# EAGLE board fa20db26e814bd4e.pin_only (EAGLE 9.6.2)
REV: C

Size 25.4 x 17.78 mm. Coordinates in mm from the lower left corner, seen from the top.
Outline: 0,15.24 0,2.54 arc90 2.54,0 22.86,0 arc90 25.4,2.54 25.4,15.24 arc90 22.86,17.78 2.54,17.78 arc90 0,15.24
Copper layers (1*16): Top 0.035mm / dielectric 1.5mm / Bottom 0.035mm
Design rules "adafruit *": minimum track width 7mil, minimum drill 15.5mil, track to track 7mil, track to pad 7mil, pad to pad 7mil, via to via 7mil, smd to smd 7mil, copper to edge 10mil, drill to drill 8mil, minimum pad ring 10mil, minimum via ring 8mil, stop-mask expansion 2mil, vias tented up to drill 20mil, thermal gap 10mil
Net classes: 1 highpower: width 0.406 mm, drill 0.483 mm; 2 lowpower: width 0.305 mm, drill 0.483 mm
tRestrict: area 11.6,7.9 to 13.5,9.9
bRestrict: area 11.1,7.4 to 14,10.4

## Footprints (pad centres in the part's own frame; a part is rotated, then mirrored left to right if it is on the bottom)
0603-NO = smd 1.075 x 1: 1 -0.85,0; 2 0.85,0
0805-NO = smd 1.24 x 1.5: 1 -0.95,0; 2 0.95,0
JST_SH4 = smd 0.6 x 1.55: 1 -1.5,2.514; 2 -0.5,2.514; 3 0.5,2.514; 4 1.5,2.514 | smd 1.2 x 1.8: MT1 -2.8,-1.386; MT2 2.8,-1.386
CHIPLED_0603_NOOUTLINE = smd 0.8 x 0.8: A 0,-0.75; C 0,0.75
SOD-323_MINI = smd 0.9 x 0.8: A 1.07,0; C -1.07,0
FIDUCIAL_1MM = smd 1 x 1: 1 0,0
1X06_ROUND_70 = drill 1 pad 1.778: 1 -6.35,0; 2 -3.81,0; 3 -1.27,0; 4 1.27,0; 5 3.81,0; 6 6.35,0
SOT363 = smd 0.5 x 0.5: 1 -0.75,-0.9; 3 0.75,-0.9; 4 0.75,0.9; 6 -0.75,0.9 | smd 0.4 x 0.5: 2 0,-0.9; 5 0,0.9
RESPACK_4X0603 = smd 0.45 x 0.9: 1 -1.3,-0.85; 2 -0.4,-0.85; 3 0.4,-0.85; 4 1.3,-0.85; 5 1.3,0.85; 6 0.4,0.85; 7 -0.4,0.85; 8 -1.3,0.85
SOLDERJUMPER_ARROW_NOPASTE = smd 0.762 x 1.524: 1 -1.016,0; 2 1.016,0
SOT23-5 = smd 0.55 x 1.2: 1 -0.95,-1.3; 2 0,-1.3; 3 0.95,-1.3; 4 0.95,1.3; 5 -0.95,1.3
QFN24_3MM_NOEP = smd 0.55 x 0.2: 1 -1.5,1; 2 -1.5,0.6; 3 -1.5,0.2; 4 -1.5,-0.2; 5 -1.5,-0.6; 6 -1.5,-1; 13 1.5,-1; 14 1.5,-0.6; 15 1.5,-0.2; 16 1.5,0.2; 17 1.5,0.6; 18 1.5,1 | smd 0.2 x 0.55: 7 -1,-1.5; 8 -0.6,-1.5; 9 -0.2,-1.5; 10 0.2,-1.5; 11 0.6,-1.5; 12 1,-1.5; 19 1,1.5; 20 0.6,1.5; 21 0.2,1.5; 22 -0.2,1.5; 23 -0.6,1.5; 24 -1,1.5
MOUNTINGHOLE_2.5_PLATED = drill 2.5 pad 3.2: P$1 0,0

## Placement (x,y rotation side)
C3  0.1uF  [0603-NO]  11.02,12.01 180 top
C5  10uF  [0805-NO]  6.6,5.59 0 top
C6  10uF  [0805-NO]  7.87,11.81 0 top
C7  0.1uF  [0603-NO]  9.78,8.7 270 top
CONN3  STEMMA_I2C_QT  [JST_SH4]  22.86,8.89 90 top
CONN4  STEMMA_I2C_QT  [JST_SH4]  2.54,8.89 270 top
D1  RED  [CHIPLED_0603_NOOUTLINE]  3.56,12.57 90 top
D2  1n4148  [SOD-323_MINI]  19.75,12.45 270 top
FID2  FIDUCIAL_1MM  [FIDUCIAL_1MM]  1.65,9.08 0 top
FID4  FIDUCIAL_1MM  [FIDUCIAL_1MM]  23.62,8.93 0 top
JP1  [1X06_ROUND_70]  12.7,2.54 0 top
JP3  [1X06_ROUND_70]  12.7,15.24 180 top
Q2  BSS138  [SOT363]  14.73,12.19 90 top
Q3  BSS138  [SOT363]  14.99,5.71 270 top
R1  10K  [0603-NO]  10.1,5.21 0 top
R2  4.7K  [RESPACK_4X0603]  17.48,11.94 270 top
R3  10K  [RESPACK_4X0603]  17.78,7.11 90 top
R4  1K  [0603-NO]  5.46,12.45 270 top
SJ1  [SOLDERJUMPER_ARROW_NOPASTE]  17.78,11.81 270 bottom
U1  MIC5225-1.8V  [SOT23-5]  7.49,8.64 0 top
U$2  [ADAFRUIT_2.5MM]  21.34,5.78 180 top
U$12  [ADAFRUIT_3.5MM]  6.63,7.06 270 bottom
U$21  MPU-9250_ICM20948  [QFN24_3MM_NOEP]  12.57,8.89 180 top
U$38  MOUNTINGHOLE2.5  [MOUNTINGHOLE_2.5_PLATED]  2.54,15.24 0 top
U$39  MOUNTINGHOLE2.5  [MOUNTINGHOLE_2.5_PLATED]  22.86,15.24 0 top
U$41  MOUNTINGHOLE2.5  [MOUNTINGHOLE_2.5_PLATED]  2.54,2.54 0 top
U$42  MOUNTINGHOLE2.5  [MOUNTINGHOLE_2.5_PLATED]  22.86,2.54 0 top
U$45  [PCBFEAT-REV-040]  21.46,5.71 0 bottom
U$46  [STEMMAQT]  22.48,4.45 90 bottom
U$47  [STEMMAQT]  2.92,13.34 270 bottom

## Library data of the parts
C3 C5-C7 CONN3 CONN4 D1 D2 JP1 JP3 Q2 Q3 R1-R4 U1 U$2 U$12 U$45 = microbuilder
FID2 FID4 SJ1 U$38 U$39 U$41 U$42 = microbuilder; BOM: EXCLUDE
U$21 = adafruit_sensor
U$46 U$47 = silks

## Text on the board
tPlace: FS | AD | AC | G | SDO | CS | ICM20948 | on | Y | X | VIN | GND | SDA | 1V8 | SCL | INT
bPlace: 1v8 Logic | ICM20948 | ADR | 9-DoF IMU | Accel: ±2~16 g / Gyro: ±250~2000 dps / Mag: ±49 Gauss | VLogic/Vcc: 3-5VDC

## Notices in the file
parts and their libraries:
microbuilder: This work is placed in the public domain, and may be freely used for commercial and non-commercial work with the following conditions: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
